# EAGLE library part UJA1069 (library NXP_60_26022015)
LIN fail-safe system basis chip The UJA1069 fail-safe System Basis Chip (SBC) replaces basic discrete components which are common in every Electronic Control Unit (ECU) with a Local Interconnect Network (LIN) interface. The fail-safe SBC supports all networking applications which control various power and sensor peripherals by using LIN as a local sub-bus. The fail-safe SBC contains the following integrated devices: LIN transceiver compliant with LIN 2.0 and SAE J2602, and compatible with LIN 1.3 Advanced independent watchdog Dedicated voltage regulator for microcontroller Serial peripheral interface (full duplex) Local wake-up input port Inhibit/limp-home output port In addition to the advantages of integrating these common ECU functions in a single package, the fail-safe SBC offers an intelligent combination of system-speciﬁc functions such as: Advanced low-power concept Safe and controlled system start-up behavior Advanced fail-safe system behavior that prevents any conceivable deadlock Detailed status reporting on system and sub-system levels The UJA1069 is designed to be used in combination with a microcontroller and a LIN controller. The fail-safe SBC ensures that the microcontroller is always started up in a deﬁned manner. In failure situations the fail-safe SBC will maintain the microcontroller function for as long as possible, to provide full monitoring and software driven fall-back operation. The UJA1069 is designed for 14 V single power supply architectures and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
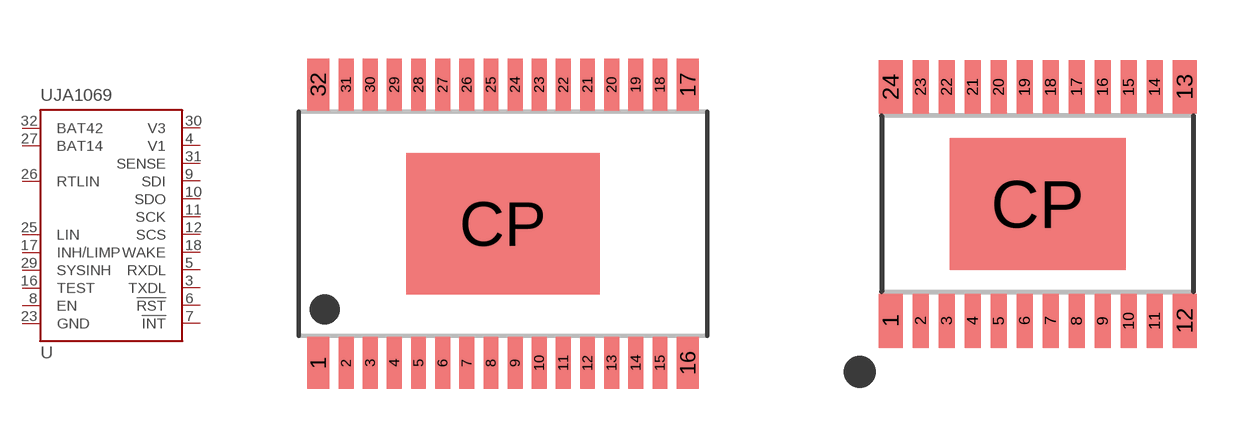
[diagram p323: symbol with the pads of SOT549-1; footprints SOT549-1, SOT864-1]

Designator prefix U

## UJA1069TW  [SOT549-1]
3  TXDL  in
4  V1  pwr
5  RXDL  out
6  !RST
7  !INT  out
8  EN  in
9  SDI
10  SDO
11  SCK
12  SCS
16  TEST  in
17  INH/LIMP  out
18  WAKE  in
23  GND  pwr
25  LIN  in
26  RTLIN  pas
27  BAT14  pwr
29  SYSINH  out
30  V3  pwr
31  SENSE  in
32  BAT42  pwr

## UJA1069TW24  [SOT864-1]
2  TXDL  in
3  V1  pwr
4  RXDL  out
5  !RST
6  !INT  out
7  EN  in
8  SDI
9  SDO
10  SCK
11  SCS
12  TEST  in
13  INH/LIMP  out
14  WAKE  in
15  GND  pwr
17  LIN  in
18  RTLIN  pas
19  BAT14  pwr
21  SYSINH  out
22  V3  pwr
23  SENSE  in
24  BAT42  pwr
CP  GND  pwr

## Footprint SOT549-1 (pad centres in mm)
SOT549-1 HTSSOP32: plastic thermal enhanced thin shrink small outline package; 32 leads;body width 6.1 mm; lead pitch 0.65 mm; exposed die pad JEDEC: MO-153 IEC: -- JEITA: --
smd 0.6 x 1.4: 1 -4.975,-3.75; 16 4.975,-3.75; 17 4.975,3.75; 32 -4.975,3.75
smd 0.4 x 1.4: 2 -4.225,-3.75; 3 -3.575,-3.75; 4 -2.925,-3.75; 5 -2.275,-3.75; 6 -1.625,-3.75; 7 -0.975,-3.75; 8 -0.325,-3.75; 9 0.325,-3.75; 10 0.975,-3.75; 11 1.625,-3.75; 12 2.275,-3.75; 13 2.925,-3.75; 14 3.575,-3.75; 15 4.225,-3.75; 18 4.225,3.75; 19 3.575,3.75; 20 2.925,3.75; 21 2.275,3.75; 22 1.625,3.75; 23 0.975,3.75; 24 0.325,3.75; 25 -0.325,3.75; 26 -0.975,3.75; 27 -1.625,3.75; 28 -2.275,3.75; 29 -2.925,3.75; 30 -3.575,3.75; 31 -4.225,3.75
smd 5.2 x 3.8: CP 0,0

## Footprint SOT864-1 (pad centres in mm)
SOT864-1 HTSSOP24: plastic thermal enhanced thin shrink small outline package; 24 leads; body width 4.4 mm; lead pitch 0.65 mm; exposed die pad JEDEC: MO-153 IEC: -- JEITA: -- NO NXP footprint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
smd 0.6 x 1.35: 1 -3.675,-2.925; 12 3.675,-2.925; 13 3.675,2.925; 24 -3.675,2.925
smd 0.4 x 1.35: 2 -2.925,-2.925; 3 -2.275,-2.925; 4 -1.625,-2.925; 5 -0.975,-2.925; 6 -0.325,-2.925; 7 0.325,-2.925; 8 0.975,-2.925; 9 1.625,-2.925; 10 2.275,-2.925; 11 2.925,-2.925; 14 2.925,2.925; 15 2.275,2.925; 16 1.625,2.925; 17 0.975,2.925; 18 0.325,2.925; 19 -0.325,2.925; 20 -0.975,2.925; 21 -1.625,2.925; 22 -2.275,2.925; 23 -2.925,2.925
smd 4.4 x 3.3: CP 0,0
